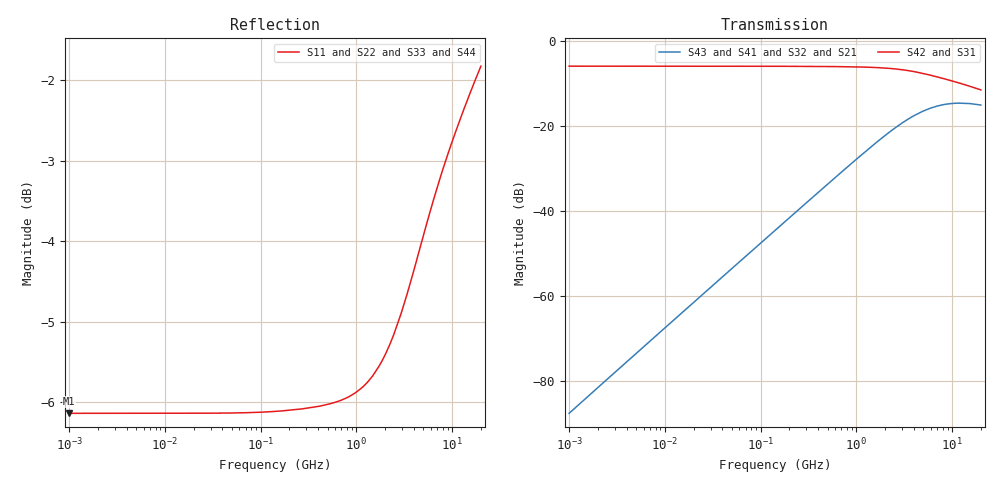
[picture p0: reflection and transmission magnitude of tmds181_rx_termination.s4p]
! Created Thu Oct 08 14:03:40 2015
# hz S db R 50
! 4 Port Network Data from SP1.SP block
! freq  dbS11  angS11  dbS12  angS12  dbS13  angS13  dbS14  angS14
!  dbS21  angS21  dbS22  angS22  dbS23  angS23  dbS24  angS24
!  dbS31  angS31  dbS32  angS32  dbS33  angS33  dbS34  angS34
!  dbS41  angS41  dbS42  angS42  dbS43  angS43  dbS44  angS44
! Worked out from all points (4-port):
!   861 points, 1 MHz to 20 GHz, reference 50 ohm
!   strongest paths, dB at 1 MHz, 11.89 MHz, 141.4 MHz, 1.682 GHz, 20 GHz:
!     S42: -5.9, -5.9, -5.9, -6.2, -11.5
!     S31: -5.9, -5.9, -5.9, -6.2, -11.5
!     S43: -87.7, -66.1, -44.6, -23.6, -15.1
!     S41: -87.7, -66.1, -44.6, -23.6, -15.1
!     S32: -87.7, -66.1, -44.6, -23.6, -15.1
!     S21: -87.7, -66.1, -44.6, -23.6, -15.1
!   lowest |S11| = -6.1 dB at 1 MHz (marker M1), VSWR 2.95, Z = 17 + j2.71e-15 ohm
!   |S11| at or under -10 dB: nowhere
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1000000  -6.14 180.0  -87.67 91.0  -5.91 0.0  -87.67 91.0
         -87.67 91.0  -6.14 180.0  -87.67 91.0  -5.91 0.0
         -5.91 0.0  -87.67 91.0  -6.14 180.0  -87.67 91.0
         -87.67 91.0  -5.91 0.0  -87.67 91.0  -6.14 180.0
2483674  -6.14 -180.0  -79.70 90.9  -5.91 -0.0  -79.70 90.9
         -79.70 90.9  -6.14 -180.0  -79.70 90.9  -5.91 -0.0
         -5.91 -0.0  -79.70 90.9  -6.14 -180.0  -79.70 90.9
         -79.70 90.9  -5.91 -0.0  -79.70 90.9  -6.14 -180.0
3.432474e8  -6.06 -177.7  -36.95 85.4  -5.96 -2.3  -36.95 85.4
            -36.95 85.4  -6.06 -177.7  -36.95 85.4  -5.96 -2.3
            -5.96 -2.3  -36.95 85.4  -6.06 -177.7  -36.95 85.4
            -36.95 85.4  -5.96 -2.3  -36.95 85.4  -6.06 -177.7
3.060799e9  -4.83 -167.1  -19.18 55.2  -6.76 -16.1  -19.18 55.2
            -19.18 55.2  -4.83 -167.2  -19.18 55.2  -6.76 -16.1
            -6.76 -16.1  -19.18 55.2  -4.83 -167.1  -19.18 55.2
            -19.18 55.2  -6.76 -16.1  -19.18 55.2  -4.83 -167.2
4.851574e9  -3.99 -165.7  -16.61 39.4  -7.56 -21.9  -16.61 39.4
            -16.61 39.4  -3.99 -165.7  -16.61 39.4  -7.56 -21.9
            -7.56 -21.9  -16.61 39.4  -3.99 -165.7  -16.61 39.4
            -16.61 39.4  -7.56 -21.9  -16.61 39.4  -3.99 -165.7
7.514986e9  -3.21 -165.9  -15.13 22.4  -8.63 -27.0  -15.13 22.4
            -15.13 22.4  -3.21 -165.9  -15.13 22.4  -8.63 -27.0
            -8.63 -27.0  -15.13 22.4  -3.21 -165.9  -15.13 22.4
            -15.13 22.4  -8.63 -27.0  -15.13 22.4  -3.21 -165.9
2e10  -1.83 -168.1  -15.06 -13.6  -11.52 -38.8  -15.06 -13.6
      -15.06 -13.6  -1.83 -168.2  -15.06 -13.6  -11.52 -38.8
      -11.52 -38.8  -15.06 -13.6  -1.83 -168.1  -15.06 -13.6
      -15.06 -13.6  -11.52 -38.8  -15.06 -13.6  -1.83 -168.2
